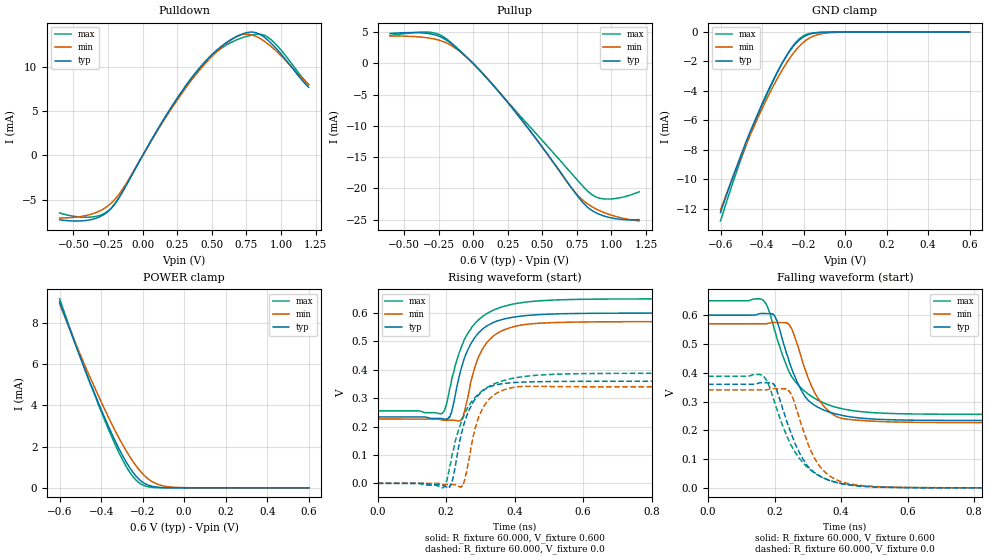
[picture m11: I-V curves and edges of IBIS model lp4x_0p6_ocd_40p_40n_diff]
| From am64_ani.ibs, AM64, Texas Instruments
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|   Model lp4x_0p6_ocd_40p_40n_diff
[Model] lp4x_0p6_ocd_40p_40n_diff
Model_type I/O
Polarity   Non-Inverting
Enable   Active-High
Vinl =  0.0V
Vinh =  0.900V
Vmeas =  0.600V
C_comp   1.772pF   1.574pF   2.047pF
[Model Spec]
Vinh   0.900V   0.900V   0.900V
Vinl   0.0V   0.0V   0.0V
Vmeas   0.600V   NA   NA
[Temperature Range]   25.000   0.125k   -40.000
[Voltage Range]   0.600V   0.570V   0.650V
[Pullup Reference]   0.600V   0.570V   0.650V
[Pulldown Reference]   0.0V   0.0V   0.0V
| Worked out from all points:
|   slope of the pulldown table from 0 to 0.09 V, typ, clamps not added: 36.7 ohm
|   slope of the pullup table from 0 to 0.09 V, typ, clamps not added: 42.8 ohm
|   GND clamp passes 1 mA (typ) near -0.25 V on its own axis
|   POWER clamp passes 1 mA (typ) near -0.26 V on its own axis
|   rising waveform, R_fixture 60.000, V_fixture 0.600: 20-80 % time 66.4ps typ, 61ps min, 80ps max; typ from 0.234 V to 0.6 V
|   rising waveform, R_fixture 60.000, V_fixture 0.0: 20-80 % time 51.3ps typ, 46.7ps min, 76.3ps max; typ from 0 V to 0.36 V
|   falling waveform, R_fixture 60.000, V_fixture 0.600: 20-80 % time 77.7ps typ, 73.1ps min, 96.8ps max; typ from 0.6 V to 0.234 V
|   falling waveform, R_fixture 60.000, V_fixture 0.0: 20-80 % time 81ps typ, 74.3ps min, 97.3ps max; typ from 0.36 V to 0 V
[Pulldown]
|Voltage   I(typ)   I(min)   I(max)
-600mV    -7.251mA   -7.047mA   -6.479mA
-392mV    -7.283mA   -6.702mA   -6.959mA
-240mV    -6.158mA   -5.537mA   -6.133mA
-145mV    -4.078mA   -3.792mA   -4.063mA
120mV     3.243mA    3.131mA    3.229mA
328mV     8.216mA    7.975mA    8.184mA
499mV     11.35mA    11.14mA    11.23mA
669mV     13.34mA    13.31mA    12.96mA
802mV     13.89mA    13.52mA    13.61mA
897mV     13.1mA     12.68mA    13.4mA
992mV     11.59mA    11.37mA    12.03mA
1.2V      7.68mA     7.991mA    7.987mA
[Pullup]
|Voltage   I(typ)   I(min)   I(max)
-600mV    4.81mA     4.404mA    4.474mA
-278mV    4.589mA    3.904mA    4.871mA
-202mV    3.866mA    3.377mA    4.097mA
-107mV    2.214mA    2.104mA    2.298mA
44.21mV   -1.008mA   -999.9uA   -1.029mA
234mV     -5.817mA   -5.774mA   -5.74mA
461mV     -12.23mA   -12.25mA   -11.38mA
707mV     -19.78mA   -19.83mA   -17.51mA
840mV     -23.26mA   -22.68mA   -20.69mA
897mV     -24.02mA   -23.4mA    -21.47mA
973mV     -24.6mA    -24.1mA    -21.72mA
1.2V      -25.02mA   -25.24mA   -20.56mA
[GND_clamp]
|Voltage   I(typ)   I(min)   I(max)
-600mV    -12.26mA   -12.07mA   -12.83mA
-535mV    -9.631mA   -9.657mA   -9.999mA
-483mV    -7.674mA   -7.84mA    -7.926mA
-457mV    -6.749mA   -6.974mA   -6.957mA
-378mV    -4.198mA   -4.571mA   -4.306mA
-326mV    -2.706mA   -3.156mA   -2.747mA
-287mV    -1.735mA   -2.22mA    -1.722mA
-248mV    -949.8uA   -1.424mA   -887.7uA
-209mV    -414uA     -806.5uA   -336.6uA
-157mV    -95.46uA   -302uA     -61.62uA
-78.26mV  -9.128uA   -53.02uA   -8.175uA
600mV     0A         0A         0A
[POWER_clamp]
|Voltage   I(typ)   I(min)   I(max)
-600mV    9.037mA    8.928mA    9.175mA
-457mV    5.197mA    5.441mA    5.166mA
-352mV    2.698mA    3.164mA    2.544mA
-313mV    1.878mA    2.4mA      1.683mA
-274mV    1.164mA    1.707mA    946.8uA
-248mV    770.4uA    1.297mA    560.4uA
-222mV    461.7uA    938.4uA    283.8uA
-196mV    245.9uA    638.9uA    120.5uA
-157mV    79.31uA    316.3uA    23.58uA
-117mV    22.67uA    136.3uA    6.088uA
-78.26mV  6.714uA    54.46uA    1.894uA
600mV     0A         0A         0A
[Ramp]
| variable   typ   min   max
dV/dt_r   0.216/51.282p   0.204/46.436p   0.233/76.119p
dV/dt_f   0.220/77.683p   0.206/72.469p   0.237/96.011p
R_load = 60.000
[Rising Waveform]
R_fixture= 60.000
V_fixture= 0.600
V_fixture_min= 0.570
V_fixture_max= 0.650
|time   V(typ)   V(min)   V(max)
0s        234.1mV    226.6mV    255.4mV
189ps     228mV      223mV      247.2mV
202ps     226.8mV    221.9mV    282.6mV
215ps     245.9mV    222.6mV    358.2mV
242ps     396mV      221.2mV    472.3mV
254ps     441.9mV    253mV      507.9mV
282ps     510.7mV    403.6mV    559.7mV
317ps     553mV      493.3mV    596.6mV
438ps     591.6mV    560.8mV    639.4mV
3ns       600mV      569.9mV    650mV
[Rising Waveform]
R_fixture= 60.000
V_fixture= 0.0
V_fixture_min= 0.0
V_fixture_max= 0.0
|time   V(typ)   V(min)   V(max)
0s        45.87uV    245uV      45.68uV
193ps     -8.225mV   -3.917mV   -13.91mV
215ps     -3.854mV   -3.411mV   84.99mV
245ps     177.4mV    -12.71mV   217.7mV
259ps     234.7mV    34.46mV    258mV
283ps     293.5mV    187.7mV    301.4mV
316ps     333.1mV    282.8mV    335.3mV
364ps     351.1mV    327.5mV    360.9mV
437ps     357.3mV    342mV      377.9mV
3ns       359.8mV    340.3mV    387.8mV
[Falling Waveform]
R_fixture= 60.000
V_fixture= 0.600
V_fixture_min= 0.570
V_fixture_max= 0.650
|time   V(typ)   V(min)   V(max)
0s        600mV      569.9mV    650mV
167ps     605.8mV    569.8mV    651mV
182ps     605.1mV    571.8mV    620.5mV
200ps     598.5mV    574.9mV    548.2mV
241ps     450.8mV    570.7mV    410.8mV
288ps     323.8mV    424.1mV    338.3mV
345ps     271.8mV    287.7mV    296.3mV
389ps     255.1mV    246.3mV    278.8mV
452ps     243.2mV    234.8mV    265.8mV
3ns       234.1mV    226.6mV    255.4mV
[Falling Waveform]
R_fixture= 60.000
V_fixture= 0.0
V_fixture_min= 0.0
V_fixture_max= 0.0
|time   V(typ)   V(min)   V(max)
0s        359.8mV    340.3mV    387.7mV
162ps     365.5mV    340.3mV    392.1mV
181ps     364.6mV    341.7mV    363.1mV
202ps     353.6mV    345mV      289.7mV
239ps     223.7mV    342.2mV    174.2mV
281ps     108.5mV    217.7mV    93.18mV
330ps     45mV       83.97mV    44.85mV
375ps     22.1mV     34.35mV    22.53mV
439ps     8.003mV    11.33mV    8.428mV
3ns       45.42uV    241.8uV    44.93uV
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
